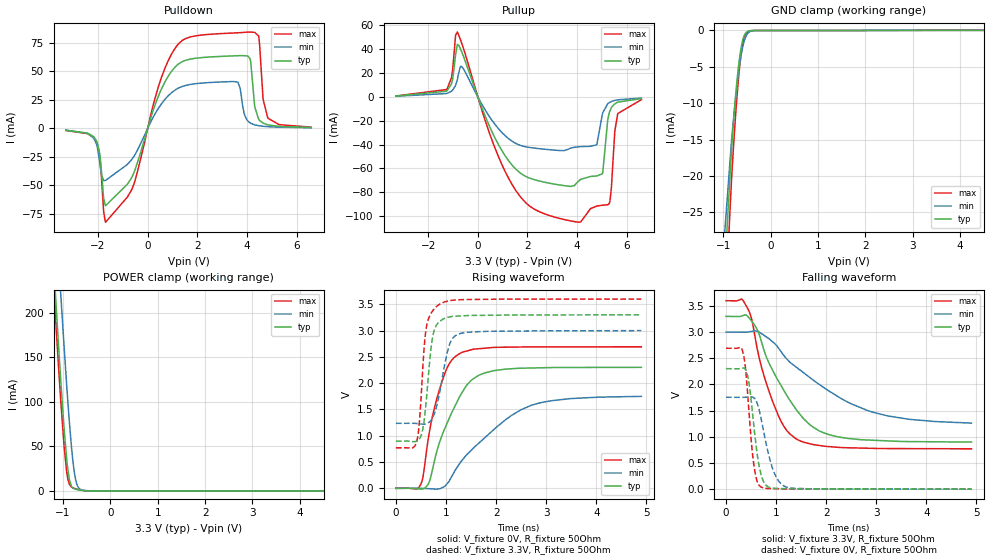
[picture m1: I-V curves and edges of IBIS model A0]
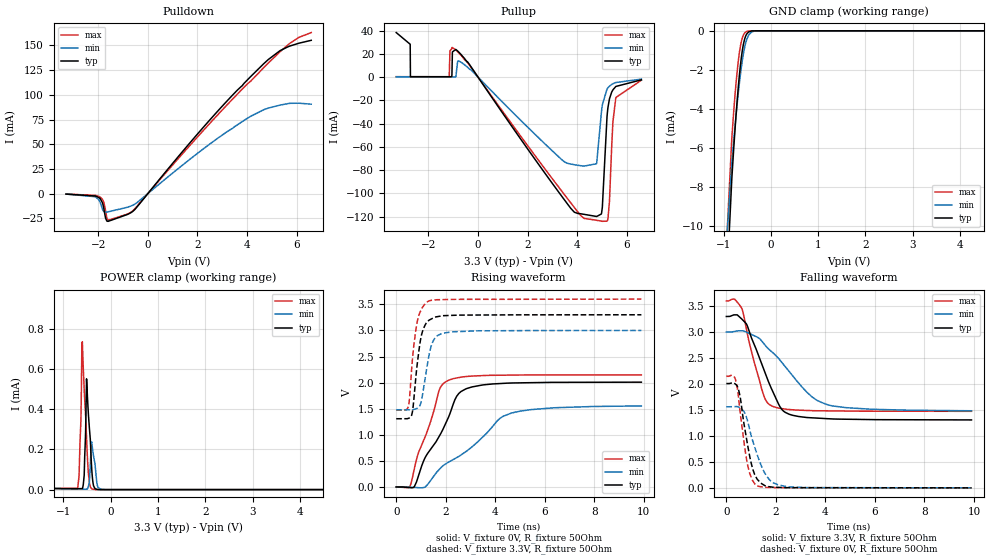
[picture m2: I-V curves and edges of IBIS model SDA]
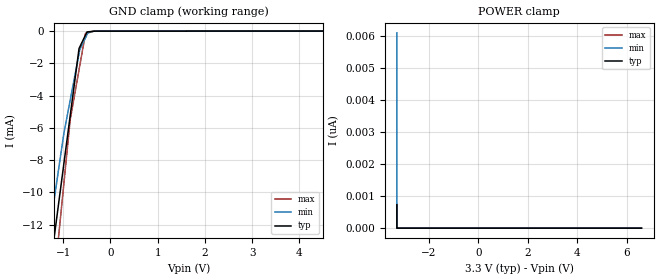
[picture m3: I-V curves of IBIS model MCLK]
| Texas Instruments Incorporated
| 25-W STEREO AMPLIFIER WITH EQ, DRC, AND DIRECT-PATH HEADPHONE AMPLIFIER
| Marketing part#   Voltage Range   Package-type   #pins/pkg drawing
| TAS5731PHP   3.0V - 3.6V   TQFP   48-pin PHP
[IBIS Ver]   4.0
[File name]   tas5731.ibs
[File Rev]   1.0
[Date]   12/06/2011
[Source]   Model built from TISPICED simulations at:
   Texas Instruments Incorporated.
   Analog-eLab, HPA
   12500 TI Blvd
   Dallas, TX -75243
   For Support e-mail: elab_ibis@list.ti.com
[Notes]   Revision History
   Rev 1.0: 12/06/2011
   - ccomp values are based on PVT settings:
   WEAK: Low Voltage, High Temperature, Weak Process
   NOM: Nominal Voltage, Nominal Temperature, Nominal Process
   STRONG: High Voltage, Low Temperature, Fast Process
   - User may change ccomp in the order of number values as
   per end simulator used
   - C_comp although listed in numberical order of value are obtained from varying PVT conditions.
   For PVT conditions for each specific value, refer to the buffer description under repective [Model].
   IBIS model user is responsible for using appropriate C_comp to simulate for Signal Integrity.
   Combined Pulldown and Pullup for SDA and A0 models are non-monotonic and reflect actual circuit behavior
   - Non-monotonic behavior in RCVR input buffer result of actual circuit behavior
   - POWER Clamp in SDIN and SDA non-monotonice as a result of circuit design
[Disclaimer] This model is designed as an aid for customers of Texas Instruments.
 TI and its licensors and suppliers make no warranties, either expressed
 or implied, with respect to this  model, including the warranties of
 merchantability or fitness for a particular purpose.
 The model is provided solely on an "as is" basis. The entire risk as to
 its quality and performance is with the customer.
[Copyright] (C)Copyright 2011 Texas Instruments Incorporated.
   All rights reserved.
|   Component TAS5731PHP
[Component]   TAS5731PHP
[Manufacturer]  Texas Instruments Incorporated
[Package]   |48-pin TQFP PHP package
|   typ   min   max
R_pkg   0.30388   0.28368   0.32548
L_pkg   1.17007nH   1.07556nH   1.26913nH
C_pkg   0.12044pF   0.11623pF   0.12502pF
[Pin] signal_name   model_name   R_pin   L_pin   C_pin
   1   NC   NC   0.02990  2.78944n  0.53700p
   2   NC   NC   0.03998  2.88166n  0.57825p
   3   NC   NC   0.02212  1.96704n  0.61220p
   4   NC   NC   0.03591  1.78508n  0.53128p
   5   NC   NC   0.05160  1.98074n  0.40003p
   6   NC   NC   0.03547  1.72704n  0.52257p
   7   NC   NC   0.00191  1.13357n  0.30728p
   8   NC   NC   0.03646  1.75364n  0.54432p
   9   NC   NC   0.05281  2.63919n  0.50765p
   10   NC   NC   0.10671  3.16224n  0.49165p
   11   NC   NC   0.03548  1.80754n  0.58303p
   12   NC   NC   0.12052  3.45688n  0.46532p
   13   NC   NC   0.05890  2.94871n  0.50957p
   14   A0/FAULT   A0   0.03496  1.78196n  0.55437p
   15   MCLK/SCLK   MCLK   0.05644  2.11672n  0.40608p
   16   NC   NC   0.02618  1.58734n  0.47778p
   17   NC   NC   0.01740  1.51281n  0.47722p
   18   NC   NC   0.02584  1.72836n  0.39928p
   19   PDNB   RESETZ   0.04720  1.88723n  0.37522p
   20   LRCLK   MCLK   0.05033  1.96369n  0.38588p
   21   NC   NC   0.05875  2.16008n  0.41013p
   22   SDIN   SDIN   0.07030  2.41824n  0.44491p
   23   SDA   SDA   0.07978  2.62752n  0.46820p
   24   SCL   SCL   0.09260  2.88018n  0.44789p
   25   RESETB   RESETZ   0.10332  3.09826n  0.43759p
   26   STEST   STEST   0.10261  3.07703n  0.47362p
   27   DVDD   POWER   0.05227  2.62143n  0.52437p
   28   DVSS   GND   0.05292  2.64171n  0.50933p
   29   NC   NC   0.13520  3.69443n  0.51281p
   30   NC   NC   0.12675  3.50374n  0.50107p
   31   NC   NC   0.11590  3.27757n  0.46113p
   32   NC   NC   0.09973  2.95872n  0.44083p
   33   NC   NC   0.10659  3.12996n  0.46056p
   34   NC   NC   0.03862  2.98539n  0.55889p
   35   NC   NC   0.04002  3.11638n  0.55699p
   36   NC   NC   0.02978  2.81881n  0.53478p
   37   NC   NC   0.04595  2.46968n  0.47620p
   38   NC   NC   0.03294  2.08092n  0.46056p
   39   NC   NC   0.03079  2.38193n  0.49542p
   40   NC   NC   0.00195  1.17956n  0.32144p
   41   NC   NC   0.00192  1.14884n  0.31347p
   42   NC   NC   0.05661  2.06401n  0.37873p
   43   NC   NC   0.05661  2.06373n  0.37877p
   44   NC   NC   0.00192  1.14932n  0.31338p
   45   NC   NC   0.00195  1.18046n  0.32271p
   46   NC   NC   0.03083  2.40701n  0.50272p
   47   NC   NC   0.03297  2.09732n  0.46601p
   48   NC   NC   0.04595  2.47080n  0.47608p
| Models and submodels in the file (7): A0 (I/O), SDA (I/O), MCLK (Input), RESETZ (Input), SCL (Input), STEST (Input), SDIN (Input)
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[Model]   A0
Model_type   I/O
Polarity   Non-Inverting
Vinl = 0.8
Vinh = 2.0
Vmeas = 1.65
Vref = 1.65
Cref = 15pF
Rref = 50
|   typ   min   max
C_comp   0.7443p   0.7440p   0.7473p
[Voltage Range]   3.3   3   3.6
[Temperature Range]   27   125   0
[Pullup Reference]   3.3   3   3.6
[Pulldown Reference]   -0   -0   -0
[Power Clamp Reference]   3.3   3   3.6
[GND Clamp Reference]   -0   -0   -0
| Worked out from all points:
|   slope of the pulldown table from 0 to 0.495 V, typ, clamps not added: 15.7 ohm
|   slope of the pullup table from 0 to 0.495 V, typ, clamps not added: 19.2 ohm
|   GND clamp passes 1 mA (typ) near -0.57 V on its own axis
|   POWER clamp passes 1 mA (typ) near -0.65 V on its own axis
|   falling waveform, V_fixture 3.3V, R_fixture 50Ohm: 20-80 % time 811ps typ, 1.47ns min, 522ps max; typ from 3.3 V to 0.899 V
|   rising waveform, V_fixture 0V, R_fixture 50Ohm: 20-80 % time 579ps typ, 1.14ns min, 377ps max; typ from 0 V to 2.3 V
|   rising waveform, V_fixture 3.3V, R_fixture 50Ohm: 20-80 % time 148ps typ, 223ps min, 128ps max; typ from 0.897 V to 3.3 V
|   falling waveform, V_fixture 0V, R_fixture 50Ohm: 20-80 % time 174ps typ, 260ps min, 141ps max; typ from 2.3 V to 0 V
[Pulldown]
|   Voltage   I(typ)   I(min)   I(max)
-3.3V     -1.623mA   -1.525mA   -1.817mA
-2.062V   -10.94mA   -13.92mA   -12.15mA
-1.696V   -67.79mA   -45.62mA   -82.24mA
-627mV    -42.42mA   -26.84mA   -52.87mA
422.4mV   27.81mA    17.28mA    35.85mA
1.155V    54.84mA    34.3mA     71.78mA
3.61V     63.69mA    40.63mA    83.79mA
4.036V    63.43mA    6.497mA    84.39mA
4.471V    8.001mA    2.345mA    80.95mA
4.65V     4.591mA    1.839mA    25.59mA
4.848V    3.066mA    1.48mA     8.894mA
6.59V     752.9uA    535.7uA    1.094mA
[GND Clamp]
|   Voltage   I(typ)   I(min)   I(max)
-3.3V     -1.551A    -1.405A    -1.594A
-1.171V   -56mA      -45.46mA   -66.77mA
-825mV    -16.3mA    -15.14mA   -20.45mA
-775.5mV  -11.9mA    -11.65mA   -15.17mA
-726mV    -8.044mA   -8.507mA   -10.47mA
-686.4mV  -5.443mA   -6.289mA   -7.237mA
-646.8mV  -3.36mA    -4.389mA   -4.571mA
-607.2mV  -1.849mA   -2.851mA   -2.569mA
-567.6mV  -895.5uA   -1.703mA   -1.257mA
-478.5mV  -126uA     -388.1uA   -168.9uA
-270.6mV  -19.24uA   -14.79uA   -27.02uA
6.59V     0A         0A         0A
[Pullup]
|   Voltage   I(typ)   I(min)   I(max)
-3.3V     660.5uA    526.6uA    750.8uA
-1.251V   5.021mA    2.888mA    6.511mA
-1.013V   14.72mA    5.612mA    22.97mA
-825mV    43.95mA    14.51mA    54.28mA
-636.9mV  37.04mA    25.19mA    44.25mA
1.492V    -59.72mA   -38.56mA   -77.2mA
4.036V    -71.05mA   -41.88mA   -105mA
4.788V    -66.29mA   -40.2mA    -91.58mA
5.016V    -64.51mA   -14.91mA   -90.81mA
5.293V    -13.68mA   -4.886mA   -89.46mA
5.64V     -4.42mA    -2.489mA   -13.99mA
6.59V     -1.469mA   -1.032mA   -2.37mA
[POWER Clamp]
|   Voltage   I(typ)   I(min)   I(max)
-3.3V     2.297A     2.39A      2.274A
-1.231V   284.3mA    385mA      259.4mA
-1.102V   170.1mA    269.1mA    146.1mA
-1.043V   120.6mA    217.4mA    97.79mA
-973.5mV  68.05mA    159.3mA    48.46mA
-924mV    36.97mA    120.1mA    22.39mA
-894.3mV  22.65mA    97.82mA    12.6mA
-825mV    5.667mA    51.79mA    4.439mA
-755.7mV  2.306mA    19.3mA     2.723mA
-666.6mV  1.123mA    3.318mA    1.463mA
-468.6mV  69.68uA    162.8uA    92.65uA
6.59V     0A         0A         0A
[Ramp]
R_load = 50
|   typ   min   max
dV/dt_r   1.3808/5.76205e-10   1.04936/1.14252e-09   1.61519/3.76139e-10
dV/dt_f   1.44054/8.09573e-10   1.0428/1.46744e-09   1.69758/5.21429e-10
[Falling Waveform]
V_fixture = 3.3V
V_fixture_min = 3V
V_fixture_max = 3.6V
R_fixture = 50Ohm
C_fixture = 0F
|   Time   V(typ)   V(min)   V(max)
0s        3.3V       3V         3.6V
311.2ps   3.308V     2.998V     3.631V
435.7ps   3.296V     3.001V     3.445V
639.2ps   3.015V     3.008V     2.606V
923.9ps   2.284V     2.82V      1.691V
1.151ns   1.892V     2.557V     1.206V
1.395ns   1.527V     2.336V     964mV
1.951ns   1.075V     1.941V     821.5mV
2.902ns   935.8mV    1.479V     779.9mV
4.9ns     899.1mV    1.262V     770.7mV
[Rising Waveform]
V_fixture = 0V
V_fixture_min = 0V
V_fixture_max = 0V
R_fixture = 50Ohm
C_fixture = 0F
|   Time   V(typ)   V(min)   V(max)
0s        867pV      40.83nV    646.3pV
495.3ps   -14.66mV   1.072mV    73.14mV
555ps     -4.913mV   -1.96mV    303mV
667.9ps   125.4mV    -7.82mV    1.071V
863.5ps   853.9mV    -8.887mV   1.861V
1.053ns   1.305V     121.5mV    2.349V
1.274ns   1.746V     477.4mV    2.564V
1.685ns   2.163V     885mV      2.658V
2.702ns   2.289V     1.578V     2.69V
4.9ns     2.301V     1.749V     2.692V
[Rising Waveform]
V_fixture = 3.3V
V_fixture_min = 3V
V_fixture_max = 3.6V
R_fixture = 50Ohm
C_fixture = 0F
|   Time   V(typ)   V(min)   V(max)
0s        897.3mV    1.236V     770.4mV
403.4ps   891.6mV    1.234V     853.6mV
455.6ps   925.7mV    1.229V     1.126V
511.8ps   1.026V     1.223V     1.879V
621.3ps   1.836V     1.233V     3.129V
725.3ps   2.835V     1.329V     3.365V
875ps     3.175V     1.834V     3.503V
1.058ns   3.258V     2.702V     3.568V
1.252ns   3.277V     2.936V     3.586V
4.9ns     3.3V       2.999V     3.6V
[Falling Waveform]
|Gnd
V_fixture = 0V
V_fixture_min = 0V
V_fixture_max = 0V
R_fixture = 50Ohm
C_fixture = 0F
|   Time   V(typ)   V(min)   V(max)
0s        2.302V     1.755V     2.692V
332.4ps   2.312V     1.754V     2.632V
387.3ps   2.288V     1.756V     2.316V
447.5ps   2.088V     1.762V     1.615V
555ps     1.209V     1.745V     462.7mV
621.3ps   676.6mV    1.639V     151.1mV
702.3ps   269.9mV    1.334V     39.33mV
926.2ps   21.43mV    403.1mV    10.6mV
1.204ns   8.623mV    40.95mV    4.629mV
4.9ns     53.1uV     297.3uV    13.79uV
[Model]   SDA
Model_type   I/O
Polarity   Non-Inverting
Vinl = 0.8
Vinh = 2.0
Vmeas = 1.65
Vref = 1.65
Cref = 15pF
Rref = 50
|   typ   min   max
C_comp   0.7443p   0.7440p   0.7473p
[Voltage Range]   3.3   3   3.6
[Temperature Range]   27   125   0
[Pullup Reference]   3.3   3   3.6
[Pulldown Reference]   -0   -0   -0
[Power Clamp Reference]   3.3   3   3.6
[GND Clamp Reference]   -0   -0   -0
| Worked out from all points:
|   slope of the pulldown table from 0 to 0.495 V, typ, clamps not added: 32.5 ohm
|   slope of the pullup table from 0 to 0.495 V, typ, clamps not added: 31.9 ohm
|   GND clamp passes 1 mA (typ) near -0.60 V on its own axis
|   POWER clamp passes 1 mA (typ) near -3.29 V on its own axis
|   falling waveform, V_fixture 3.3V, R_fixture 50Ohm: 20-80 % time 1.01ns typ, 1.72ns min, 668ps max; typ from 3.3 V to 1.31 V
|   rising waveform, V_fixture 0V, R_fixture 50Ohm: 20-80 % time 1.29ns typ, 2.35ns min, 888ps max; typ from 0 V to 2.01 V
|   rising waveform, V_fixture 3.3V, R_fixture 50Ohm: 20-80 % time 299ps typ, 342ps min, 283ps max; typ from 1.31 V to 3.3 V
|   falling waveform, V_fixture 0V, R_fixture 50Ohm: 20-80 % time 440ps typ, 642ps min, 368ps max; typ from 2.01 V to 0 V
[Pulldown]
|   Voltage   I(typ)   I(min)   I(max)
-3.3V     -559.9uA   -542.7uA   -469.7uA
-2.122V   -2.468mA   -3.204mA   -1.888mA
-1.983V   -3.945mA   -6.17mA    -2.853mA
-1.785V   -14.05mA   -17.97mA   -8.449mA
-1.706V   -24.93mA   -18.84mA   -17.74mA
-1.637V   -28.06mA   -18.67mA   -26.01mA
-686.4mV  -19.39mA   -12.65mA   -19.01mA
2.363V    70.7mA     47.61mA    67.34mA
4.155V    118.7mA    78.38mA    114mA
5.333V    144.8mA    89.61mA    143.7mA
6.095V    152.3mA    91.5mA     158.2mA
6.59V     155.2mA    90.54mA    163.1mA
[GND Clamp]
|   Voltage   I(typ)   I(min)   I(max)
-3.3V     -1.514A    -1.357A    -1.56A
-1.607V   -47.21mA   -35.03mA   -43.52mA
-825mV    -7.581mA   -6.783mA   -5.501mA
-745.8mV  -4.664mA   -4.596mA   -2.961mA
-706.2mV  -3.403mA   -3.61mA    -1.948mA
-666.6mV  -2.316mA   -2.718mA   -1.15mA
-627mV    -1.437mA   -1.937mA   -591.7uA
-587.4mV  -790.1uA   -1.288mA   -259.8uA
-508.2mV  -156.3uA   -434.6uA   -32.58uA
-409.2mV  -10.58uA   -65.64uA   -1.24uA
-270.6mV  -46.46nA   -2.385uA   0A
6.59V     0A         0A         0A
[Pullup]
|   Voltage   I(typ)   I(min)   I(max)
-3.3V     38.34mA    165.8uA    389.7uA
-2.736V   28.28mA    154uA      344uA
-2.726V   348.7uA    153.8uA    343.5uA
-1.162V   326.1uA    144.3uA    317.2uA
-1.063V   357.5uA    144.2uA    24.35mA
-894.3mV  23.79mA    154.1uA    23.32mA
4.026V    -117.4mA   -75.91mA   -116mA
4.778V    -119.9mA   -74.6mA    -123.2mA
4.976V    -117.8mA   -30.66mA   -124mA
5.224V    -29.62mA   -9.709mA   -123.2mA
5.561V    -8.046mA   -4.65mA    -17.58mA
6.59V     -2.35mA    -1.735mA   -2.682mA
[POWER Clamp]
|   Voltage   I(typ)   I(min)   I(max)
-3.3V     1.038mA    9.254mA    692.2uA
-2.874V   479.6uA    1.182mA    323.7uA
-2.627V   255.8uA    434.3uA    140.4uA
-2.023V   7.025uA    93.11uA    6.497uA
-696.3mV  4.878uA    2.32uA     6.22uA
-627mV    4.868uA    2.316uA    346.2uA
-597.3mV  4.824uA    2.315uA    736.5uA
-557.7mV  72.19uA    2.312uA    496.7uA
-508.2mV  551.7uA    2.308uA    257.9uA
-389.4mV  71.88uA    217.3uA    3.215uA
-211.2mV  69.71nA    2.032uA    0A
6.59V     0A         0A         0A
[Ramp]
R_load = 50
|   typ   min   max
dV/dt_r   1.20505/1.28979e-09   0.932073/2.35176e-09   1.28889/8.87513e-10
dV/dt_f   1.1951/1.01652e-09   0.909529/1.72053e-09   1.27543/6.67234e-10
[Falling Waveform]
V_fixture = 3.3V
V_fixture_min = 3V
V_fixture_max = 3.6V
R_fixture = 50Ohm
C_fixture = 0F
|   Time   V(typ)   V(min)   V(max)
0s        3.3V       3V         3.6V
332.3ps   3.331V     3.012V     3.634V
631.3ps   3.247V     3.024V     3.448V
830.9ps   3.138V     2.994V     3.012V
1.472ns   2.334V     2.803V     1.834V
1.851ns   1.881V     2.614V     1.574V
2.371ns   1.456V     2.339V     1.517V
3.451ns   1.349V     1.755V     1.487V
4.086ns   1.332V     1.601V     1.483V
9.9ns     1.308V     1.484V     1.474V
[Rising Waveform]
V_fixture = 0V
V_fixture_min = 0V
V_fixture_max = 0V
R_fixture = 50Ohm
C_fixture = 0F
|   Time   V(typ)   V(min)   V(max)
0s        951pV      57.66nV    -337.4nV
565.5ps   -13.03mV   -3.808mV   23.65mV
730.3ps   4.516mV    -8.506mV   343.5mV
1.146ns   541.2mV    -6.853mV   936.5mV
1.742ns   976.2mV    337.4mV    1.863V
2.078ns   1.301V     466.5mV    2.037V
2.371ns   1.673V     543.9mV    2.083V
2.615ns   1.828V     613.4mV    2.105V
4.634ns   1.992V     1.413V     2.144V
9.9ns     2.008V     1.553V     2.148V
[Rising Waveform]
V_fixture = 3.3V
V_fixture_min = 3V
V_fixture_max = 3.6V
R_fixture = 50Ohm
C_fixture = 0F
|   Time   V(typ)   V(min)   V(max)
0s        1.308V     1.479V     1.474V
467.9ps   1.312V     1.478V     1.512V
541.1ps   1.326V     1.477V     1.722V
622.6ps   1.374V     1.48V      2.249V
816.5ps   2.216V     1.502V     3.08V
984.4ps   2.827V     1.593V     3.372V
1.318ns   3.193V     2.506V     3.564V
1.541ns   3.25V      2.838V     3.583V
2.058ns   3.286V     2.96V      3.593V
9.9ns     3.3V       3V         3.6V
[Falling Waveform]
|Gnd
V_fixture = 0V
V_fixture_min = 0V
V_fixture_max = 0V
R_fixture = 50Ohm
C_fixture = 0F
|   Time   V(typ)   V(min)   V(max)
0s        2.009V     1.56V      2.148V
325.6ps   2.014V     1.564V     2.132V
475.2ps   1.918V     1.56V      1.812V
715ps     1.228V     1.467V     874.5mV
849.4ps   850.4mV    1.304V     465.1mV
1.047ns   395.2mV    934.3mV    155.2mV
1.256ns   160.8mV    625.9mV    37.79mV
1.755ns   20.76mV    150.1mV    8.108mV
2.528ns   3.802mV    17.6mV     2.766mV
9.9ns     21.89uV    142.1uV    -337.4nV
[Model]   MCLK
Model_type   Input
Vinl = .8
Vinh = 2
|   typ   min   max
C_comp   0.7443p   0.7440p   0.7473p
[Voltage Range]   3.3   3   3.6
[Temperature Range]   27   125   0
[Power Clamp Reference]   3.3   3   3.6
[GND Clamp Reference]   -0   -0   -0
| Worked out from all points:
|   GND clamp passes 1 mA (typ) near -0.65 V on its own axis
[GND Clamp]
|   Voltage   I(typ)   I(min)   I(max)
-3.3V     -1.514A    -1.357A    -1.56A
-1.441V   -19.09mA   -15.41mA   -22.82mA
-1.238V   -13.78mA   -11.35mA   -16.83mA
-988.3mV  -8.243mA   -6.357mA   -9.481mA
-852.9mV  -5.236mA   -4.277mA   -5.487mA
-665.8mV  -1.08mA    -1.402mA   -2.396mA
-649.3mV  -979.8uA   -1.149mA   -2.125mA
-529.9mV  -249.7uA   -419.5uA   -152.6uA
-497.8mV  -53.24uA   -223uA     -123.4uA
-358.6mV  -12.14uA   -10.45uA   -5.776uA
-237.4mV  -3.461uA   -2.36uA    -4.816uA
6.6V      0A         0A         0A
[POWER Clamp]
|   Voltage   I(typ)   I(min)   I(max)
-3.3V     728.6pA    6.099nA    754.7pA
-3.3V     0A         0A         0A
-3.3V     0A         0A         0A
6.6V      0A         0A         0A
